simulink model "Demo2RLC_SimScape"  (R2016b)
settings: Solver=ode23s  StartTime=0.0  StopTime=20  RelTol=1e-10  EnableMultiTasking=on
libraries: fl_lib x6, nesl_utility x3, elec_lib x1

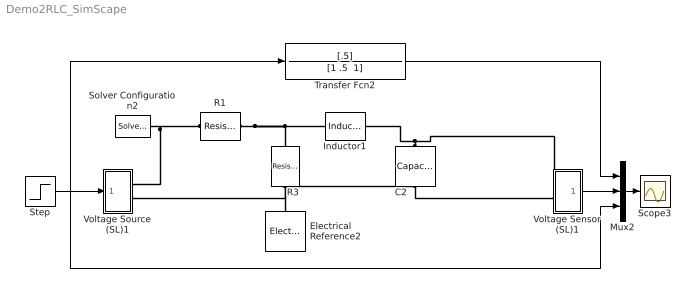
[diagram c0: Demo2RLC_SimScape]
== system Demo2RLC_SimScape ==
  C2 : fl_lib/Electrical/Electrical Elements/Capacitor  c=1 F  r=0 Ohm  g=0 1/Ohm  i_specify=off  i_priority=None  i=0 A  v_specify=off  v_priority=None  v=0 V  vc_specify=on  vc_priority=High  vc=0 V
  Electrical Reference2 : fl_lib/Electrical/Electrical Elements/Electrical Reference
  Inductor1 : elec_lib/Passive Devices/Inductor  l=1 H  L_tol=20  enable_L_tol=0  tol_distribution=1  nSigma=4  r=0 Ohm  g=1e-9 1/Ohm  initI=0 A  enable_operating_limits=0  operating_limit_action=2  max_working_current=1 A  power_rating=1 W  enable_faults=0  fault_action=1  lambdaPercent=50  k_faulted=0.9999 Ohm  turnsShort=0  openCct=0  groundShort=0  groundShortG=0 1/Ohm  tau_fault=0.001 s  enable_temporal_fault=0  t_fault=1 s  enable_behavioral_fault=0  max_permissible_voltage=100 V  n_fail_on_voltage=1  max_permissible_current=1 A  t_fail_on_current=1 s
  Mux2 : Mux  Inputs=3
  R1 : fl_lib/Electrical/Electrical Elements/Resistor  R=1 Ohm  i_specify=off  i_priority=None  i=0 A  v_specify=off  v_priority=None  v=0 V
  R3 : fl_lib/Electrical/Electrical Elements/Resistor  R=1 Ohm  i_specify=off  i_priority=None  i=0 A  v_specify=off  v_priority=None  v=0 V
  Scope3 : Scope
  Solver Configuration2 : nesl_utility/Solver Configuration  PhysicalDomain=network_engine_domain  SubClassName=solver  LeftPortType=input  RightPortType=generic  Accelerate=off  Tones=[]  Harmonics=[]  SimulateNoise=off  Profile=off  UseLocalSampling=off  EnableSwitchedLinearOptims=on  FrequencyDomain=off  UseCCode=off  RelTol=0.001  AbsTol=1e-06  MinStep=1e-09  ToWorkspace=off  RevertToSquareIcSolve=off  NumHomotopyIterations=100  PhasorMode=off  PhasorModeNumHarmonics=1  OverrideAbsTol=off  DoDC=off  ResidualTolerance=1e-6  UseLocalSolver=off  LocalSolverChoice=NE_TRAPEZOIDAL_ADVANCER  LocalSolverSampleTime=.0001  DoFixedCost=off  MaxNonlinIter=3  MaxModeIter=2  LinearAlgebra=Sparse  DelaysMemoryBudget=1024  AutomaticFiltering=on  FilteringTimeConstant=0.001
  Step : Step  SampleTime=0
  Transfer Fcn2 : TransferFcn  Numerator=[.5]  Denominator="[1 .5  1]"
  Voltage Sensor (SL)1 : Subsystem
  Voltage Source (SL)1 : Subsystem
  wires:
  Mux2/1 -> Scope3/1
  Step/1 -> Transfer Fcn2/1, Mux2/3, Voltage Source (SL)1/1(S)
  Voltage Sensor (SL)1/1(v) -> Mux2/2
  Transfer Fcn2/1 -> Mux2/1
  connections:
  R1/RConn1 -- Inductor1/LConn1 -- R3/LConn1
  Voltage Source (SL)1/RConn1 -- R1/LConn1 -- Solver Configuration2/RConn1
  C2/RConn1 -- Voltage Source (SL)1/RConn2 -- Electrical Reference2/LConn1 -- R3/RConn1 -- Voltage Sensor (SL)1/LConn2
  C2/LConn1 -- Inductor1/RConn1 -- Voltage Sensor (SL)1/LConn1

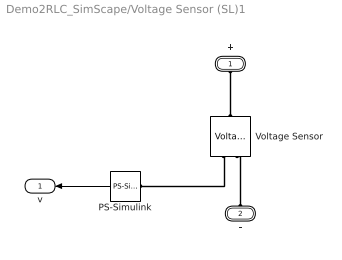
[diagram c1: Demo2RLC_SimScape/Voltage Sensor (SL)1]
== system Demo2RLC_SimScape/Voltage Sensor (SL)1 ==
  PS-Simulink : nesl_utility/PS-Simulink Converter  PhysicalDomain=network_engine_domain  SubClassName=ps_output  LeftPortType=input  RightPortType=output  PseudoPeriodic=off  Frequencies=[]  Unit=V  AffineConversion=off
  Voltage Sensor : fl_lib/Electrical/Electrical Sensors/Voltage Sensor
  + : PMIOPort  Port=1  Side=Left
  - : PMIOPort  Port=2  Side=Left
  v : Outport
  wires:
  PS-Simulink/1 -> v/1
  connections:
  Voltage Sensor/RConn1 -- PS-Simulink/LConn1
  +/RConn1 -- Voltage Sensor/LConn1
  -/RConn1 -- Voltage Sensor/RConn2

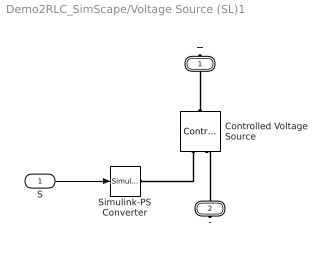
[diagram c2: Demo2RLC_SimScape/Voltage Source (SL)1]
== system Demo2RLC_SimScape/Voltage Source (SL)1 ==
  S : Inport
  Controlled Voltage Source : fl_lib/Electrical/Electrical Sources/Controlled Voltage Source
  Simulink-PS Converter : nesl_utility/Simulink-PS Converter  PhysicalDomain=network_engine_domain  SubClassName=ps_input  LeftPortType=input  RightPortType=output  PseudoPeriodic=off  Frequencies=[]  NoiseDistribution=none  NoiseParameters=[]  Unit=V  AffineConversion=off  InputFiltering=off  SimscapeFilterOrder=1  InputFilterTimeConstant=.001  UdotUserProvided=0
  + : PMIOPort  Port=1  Side=Right
  - : PMIOPort  Port=2  Side=Right
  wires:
  S/1 -> Simulink-PS Converter/1
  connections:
  Controlled Voltage Source/RConn1 -- Simulink-PS Converter/RConn1
  -/RConn1 -- Controlled Voltage Source/RConn2
  +/RConn1 -- Controlled Voltage Source/LConn1
